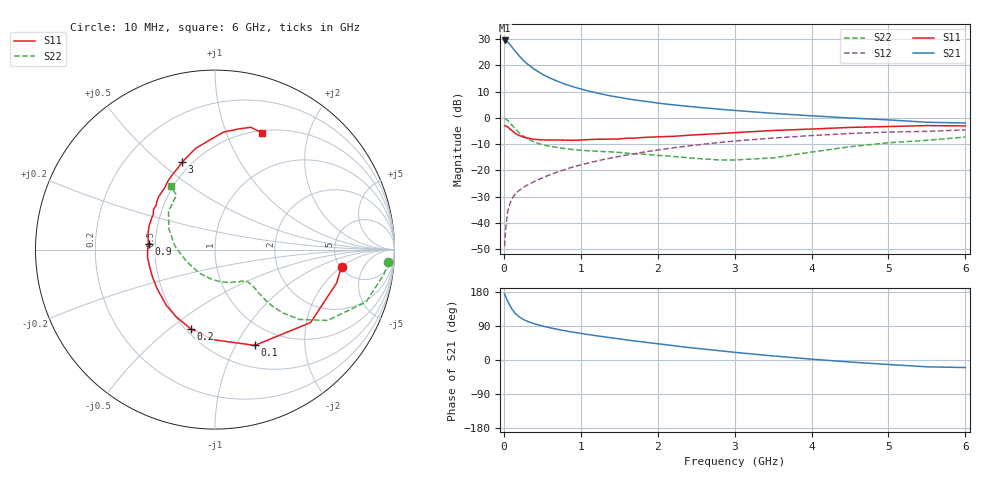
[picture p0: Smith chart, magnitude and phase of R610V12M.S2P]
! SIEMENS Small Signal Semiconductors
! BFR193
! Si NPN RF Bipolar Junction Transistor in SOT23
! VCE = 10 V  IC = 12 mA
! Common Emitter S-Parameters:  May  1996
# GHz  S  MA  R  50
!  f  S11  S21  S12  S22
! GHz  MAG  ANG  MAG  ANG  MAG  ANG  MAG  ANG
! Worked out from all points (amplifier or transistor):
!   36 points, 10 MHz to 6 GHz, reference 50 ohm
!   highest |S21| = 29.4 dB at 10 MHz (marker M1)
!   |S21| within 3 dB of that: start of sweep to 118.4 MHz
!   unconditionally stable (mu >= 1): 734.1 MHz to 2.123 GHz
!   at 250 MHz: K = 0.68, MSG = 24.3 dB, |S12| = -26.6 dB
!   at 1.4 GHz: K = 1.04, MAG = 10.6 dB, |S12| = -15.3 dB
!   at 6 GHz: K = 0.94, MSG = 1.3 dB, |S12| = -4.6 dB
!   S11 on the Smith chart (normalised r, x): 10 MHz: 5.14, -1.98; 100 MHz: 0.75, -1.20; 200 MHz: 0.53, -0.59; 900 MHz: 0.46, +0.03; 3 GHz: 0.45, +0.60; 6 GHz: 0.53, +1.35
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0.01  0.7114 -7.7  29.65 174.5  0.0036 79.0  0.9676 -4.0
0.02  0.7027 -15.3  29.44 169.0  0.0067 77.8  0.9525 -8.1
0.05  0.6702 -37.3  27.72 154.8  0.0168 73.2  0.8911 -19.1
0.1  0.578 -67.4  22.71 136.0  0.0283 64.5  0.7408 -32.2
0.15  0.5026 -90.7  18.33 122.5  0.0358 58.8  0.6124 -39.5
0.2  0.4615 -107.2  15.05 113.8  0.0415 57.7  0.5173 -43.0
0.25  0.4319 -120.2  12.53 107.4  0.0469 56.7  0.4523 -44.5
0.3  0.4124 -131.0  10.75 102.5  0.052 57.8  0.4071 -45.0
0.4  0.3891 -146.1  8.356 95.5  0.0617 60.0  0.3434 -44.8
0.5  0.3799 -156.9  6.752 89.7  0.0716 61.7  0.3068 -44.1
0.6  0.3766 -166.1  5.703 85.0  0.0825 62.6  0.2866 -43.9
0.8  0.3759 -178.9  4.342 77.0  0.104 63.5  0.2586 -44.5
0.9  0.3718 175.0  3.895 73.5  0.1158 63.9  0.2481 -45.0
1.1  0.3848 165.9  3.243 67.2  0.1383 63.5  0.2363 -48.1
1.3  0.3909 157.2  2.775 61.2  0.1615 62.3  0.2271 -51.2
1.6  0.4091 146.7  2.307 52.9  0.1961 60.2  0.2123 -58.5
2.2  0.4435 129.3  1.763 38.0  0.2675 53.9  0.184 -78.4
3  0.521 110.5  1.381 20.2  0.3611 43.3  0.1576 -122.8
3.5  0.5729 101.1  1.215 10.7  0.4115 36.0  0.1721 -157.7
4.5  0.6555 86.0  0.99 -5.3  0.5022 21.7  0.2813 155.9
5.5  0.7102 73.7  0.823 -18.0  0.5514 6.9  0.3723 125.2
6  0.7012 67.9  0.794 -19.9  0.5891 2.5  0.4303 125.1
